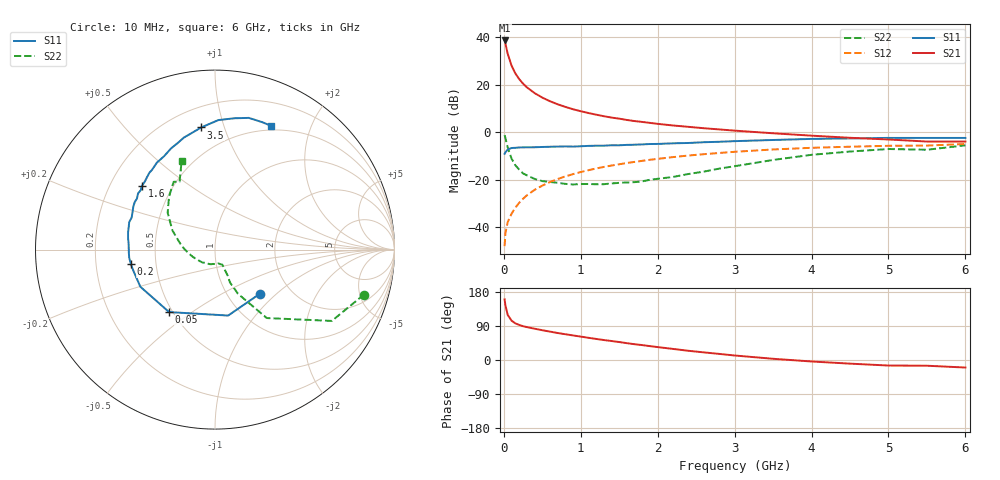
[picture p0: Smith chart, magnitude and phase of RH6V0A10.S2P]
! SIEMENS Small Signal Semiconductors
! BFR106
! Si NPN RF Bipolar Junction Transistor in SOT23
! VCE = 6 V  IC = 100 mA
! Common Emitter S-Parameters:  August  1996
# GHz  S  MA  R  50
!  f  S11  S21  S12  S22
! GHz  MAG  ANG  MAG  ANG  MAG  ANG  MAG  ANG
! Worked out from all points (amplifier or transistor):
!   36 points, 10 MHz to 6 GHz, reference 50 ohm
!   highest |S21| = 38.6 dB at 10 MHz (marker M1)
!   |S21| within 3 dB of that: start of sweep to 32.11 MHz
!   unconditionally stable (mu >= 1): 164.5 MHz to 2.474 GHz; 5.454 GHz to 5.641 GHz
!   at 250 MHz: K = 1.06, MAG = 22.7 dB, |S12| = -28.0 dB
!   at 1.4 GHz: K = 1.07, MAG = 8.4 dB, |S12| = -14.0 dB
!   at 6 GHz: K = 0.99, MSG = 0.5 dB, |S12| = -5.0 dB
!   S11 on the Smith chart (normalised r, x): 10 MHz: 1.41, -0.79; 50 MHz: 0.48, -0.41; 200 MHz: 0.36, -0.07; 1.6 GHz: 0.34, +0.34; 3.5 GHz: 0.33, +0.84; 6 GHz: 0.45, +1.46
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0.01  0.3508 -44.4  84.99 160.0  0.004 77.8  0.867 -16.8
0.02  0.3747 -78.7  73.46 144.7  0.0075 66.4  0.7627 -31.4
0.05  0.4319 -126.3  44.8 119.2  0.0128 60.3  0.4781 -52.9
0.1  0.4644 -153.5  25.18 103.9  0.0192 65.4  0.2776 -62.5
0.15  0.4691 -164.8  17.18 96.6  0.0259 68.2  0.201 -65.5
0.2  0.476 -170.2  13.05 92.5  0.0328 71.0  0.1631 -64.0
0.25  0.4801 -174.6  10.48 89.2  0.0398 71.9  0.1358 -64.1
0.3  0.4804 -178.0  8.769 86.8  0.047 73.3  0.1236 -64.4
0.4  0.4817 176.7  6.638 82.6  0.0612 74.1  0.1038 -64.0
0.5  0.4883 172.6  5.333 78.6  0.0751 73.4  0.0935 -64.0
0.6  0.4937 168.8  4.474 74.9  0.0896 73.0  0.0897 -66.6
0.7  0.4974 165.0  3.858 71.2  0.1033 72.1  0.0862 -70.4
0.9  0.4975 159.0  3.035 64.8  0.1312 69.6  0.0795 -76.4
1.1  0.5146 152.1  2.527 58.6  0.1587 67.1  0.0812 -87.6
1.3  0.5197 146.8  2.166 52.7  0.1855 64.2  0.0805 -97.7
1.6  0.5405 138.8  1.805 44.4  0.2247 60.0  0.0875 -115.7
2.2  0.5831 123.7  1.383 29.2  0.2991 51.1  0.1144 -151.0
2.8  0.6282 109.5  1.142 16.1  0.3653 41.8  0.1713 178.7
3.5  0.6851 96.4  0.948 3.2  0.4329 31.3  0.2605 155.7
4.5  0.7397 81.6  0.762 -9.6  0.4944 16.5  0.3911 130.9
5.5  0.7573 69.5  0.635 -15.1  0.5224 6.7  0.4271 117.5
6  0.7568 65.5  0.634 -19.9  0.5638 -0.3  0.5284 110.6
